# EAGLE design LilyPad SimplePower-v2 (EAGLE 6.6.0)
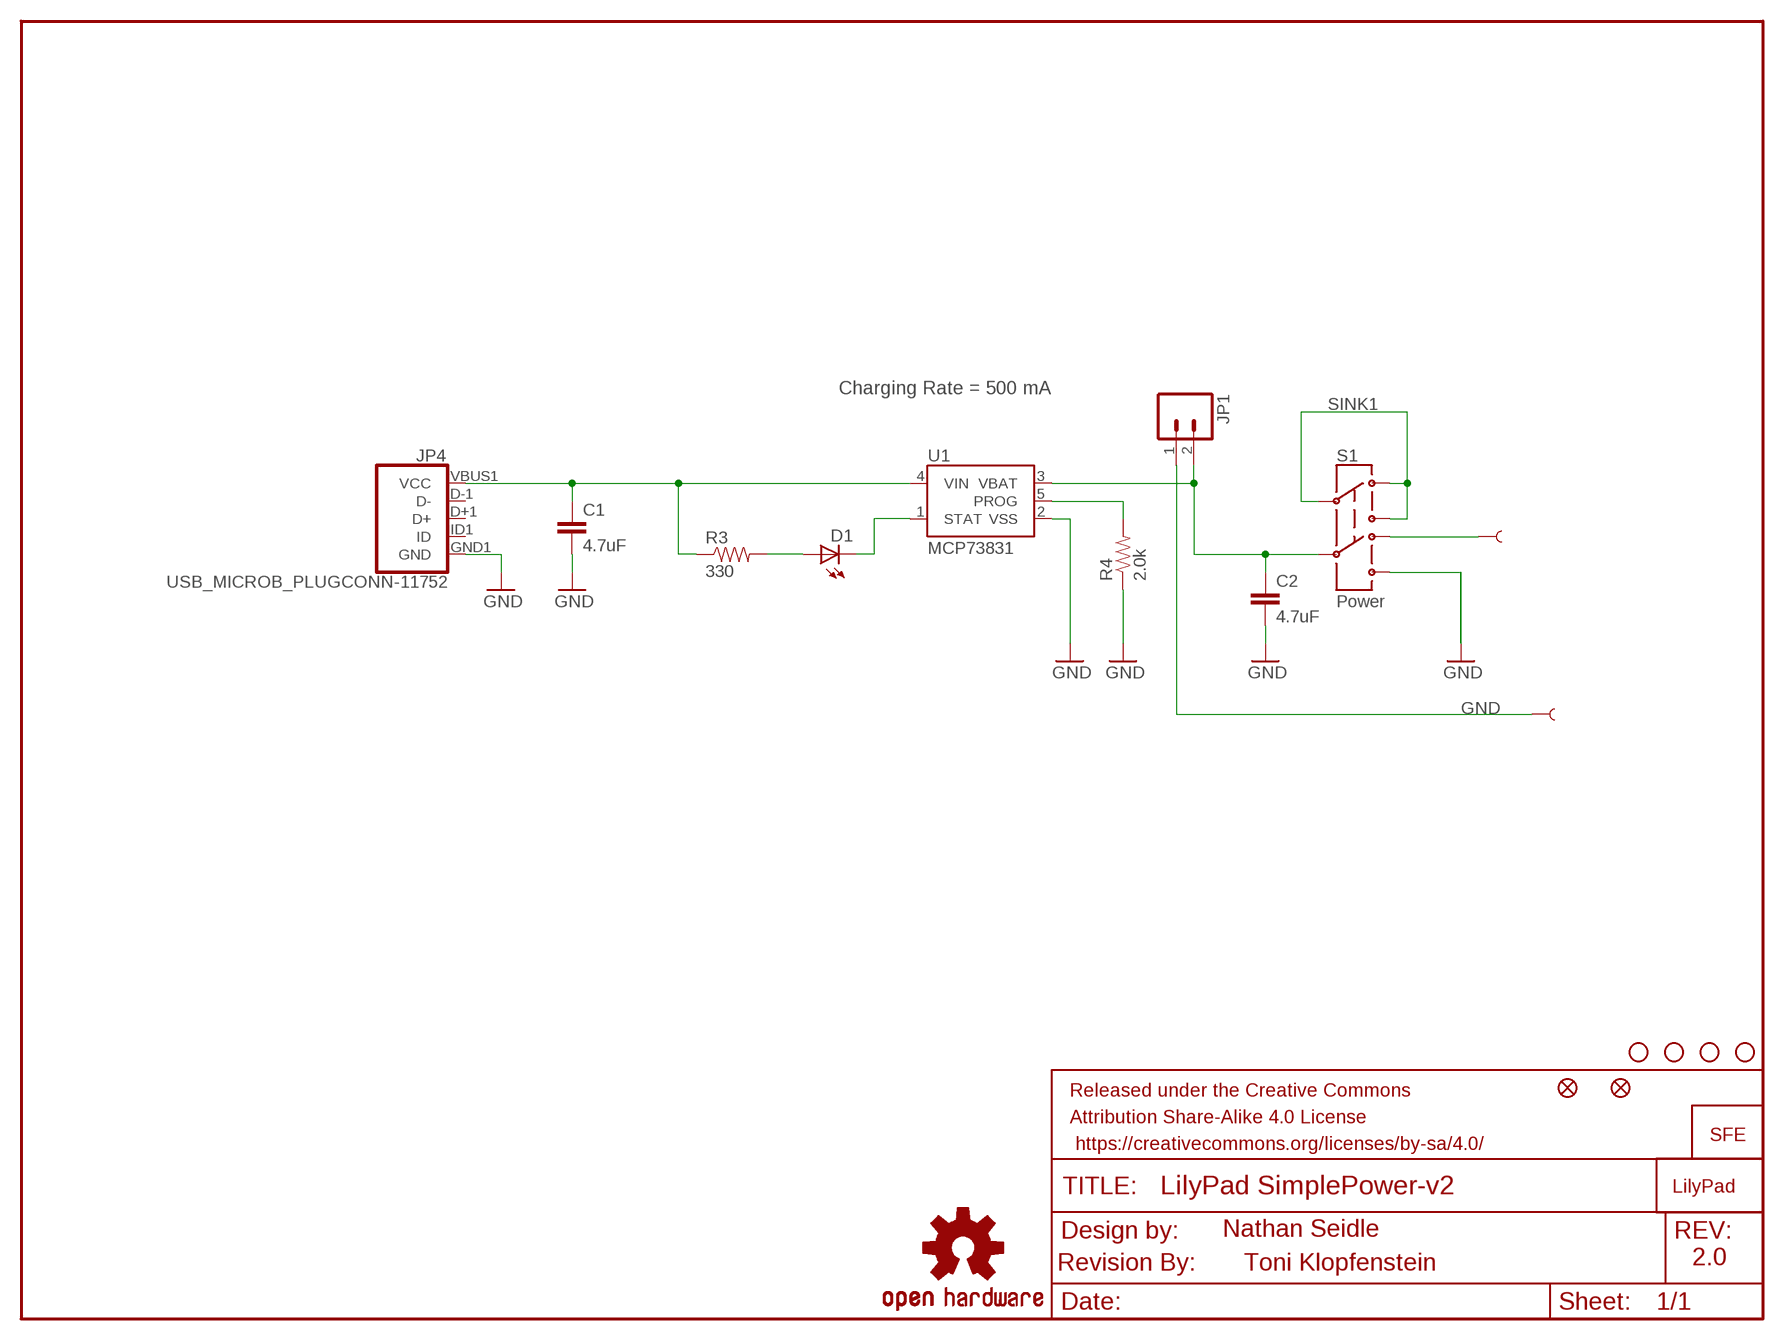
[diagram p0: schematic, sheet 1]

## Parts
C1  4.7uF  4.7UF-6.3V-10%(0603)0603  [0603-CAP]
C2  4.7uF  4.7UF-6.3V-10%(0603)0603  [0603-CAP]
D1  LED-YELLOW0603  [LED-0603]
FID1  FIDUCIAL1X2  [FIDUCIAL-1X2]
FID2  FIDUCIAL1X2  [FIDUCIAL-1X2]
FRAME1  FRAME-LETTER  [CREATIVE_COMMONS]
JP1  M02-JST-2MM-SMT  [JST-2-SMD]
JP3  LOGO-SFESK  [SFE-LOGO-FLAME]
JP4  USB_MICROB_PLUGCONN-11752  [USB-B-MICRO-SMD_V03]
R3  330  330OHM1/10W1%(0603)  [0603-RES]
R4  2.0k  2.0KOHM1/10W5%(0603)  [0603-RES]
S1  Power  SWITCH-DPDTSMD  [AYZ0202]
STANDOFF1  SEW-HOLE-NO-PAD  [SEW-HOLE-NO-PAD]
STANDOFF2  SEW-HOLE-NO-PAD  [SEW-HOLE-NO-PAD]
STANDOFF3  SEW-HOLE-NO-PAD  [SEW-HOLE-NO-PAD]
STANDOFF4  SEW-HOLE-NO-PAD  [SEW-HOLE-NO-PAD]
U1  MCP73831  [SOT23-5]
U$1  LOGO-LPLP  [LOGO-LILYPAD]
U$3  SEWTAP9  [PETAL-LONG-1-2SIDE]
U$4  SEWTAP9  [PETAL-LONG-1-2SIDE]
U$5  OSHW-LOGOS  [OSHW-LOGO-S]
U$6  REVISION  [REVISION]

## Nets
GND: C1.2 C2.2 JP1.1 JP4.GND1(GND) R4.1 S1.6 U1.2(VSS) U$3.1
N$1: C2.1 JP1.2 S1.5 U1.3(VBAT)
N$3: C1.1 JP4.VBUS1(VCC) R3.1 U1.4(VIN)
N$4: D1.C U1.1(STAT)
N$5: D1.A R3.2
N$6: S1.4 U$4.1
N$7: R4.2 U1.5(PROG)
SINK1: S1.1 S1.2 S1.3
Unconnected: JP4.D+1(D+) JP4.D-1(D-) JP4.ID1(ID)

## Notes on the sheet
- Charging Rate = 500 mA
- Nathan Seidle
- Toni Klopfenstein | 2.0

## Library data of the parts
C1 C2 = SparkFun-Capacitors:4.7UF-6.3V-10%(0603): CAP-08280; PROD_ID: CAP-08280
D1 = SparkFun-LED:LED-YELLOW: Yellow SMD LEDs; PROD_ID: DIO-09003
FID1 FID2 = SparkFun-Aesthetics:FIDUCIAL: Fiducial Alignment Points
FRAME1 = SparkFun-Aesthetics:FRAME-LETTER: Schematic Frame
JP1 = SparkFun:M02: Header 2
JP3 = SparkFun-Aesthetics:LOGO-SFE: Spark Fun Electronics PCB Logo
JP4 = SparkFun-Connectors:USB_MICROB_PLUG: USB Micro-B Plug Comes in a variety of packages. Check out Hirose's ZX-x0 line: http://www.hirose.co.jp/cataloge_hp/e24200011.pdf; PROD_ID: CONN-11752
R3 = SparkFun-Resistors:330OHM1/10W1%(0603): RES-00818; PROD_ID: RES-00818
R4 = SparkFun-Resistors:2.0KOHM1/10W5%(0603): RES-08296; PROD_ID: RES-08296
S1 = SparkFun:SWITCH-DPDT: DPDT Version of the COM-00597
STANDOFF1-STANDOFF4 = Local Library:SEW-HOLE-NO-PAD: #4 Stand Off
U1 = SparkFun-PowerIC:MCP73831: Miniature single cell, fully integrated Li-Ion, Li-polymer charge management controller http://ww1.microchip.com/downloads/en/DeviceDoc/21984a.pdf IC-09995; PROD_ID: IC-09995
U$1 = LilyPad-Wearables:LOGO-LP
U$3 U$4 = LilyPad-Wearables:SEWTAP
U$5 = SparkFun-Aesthetics:OSHW-LOGO: Open Source Hardware Logo This logo indicates the piece of hardware it is found on incorporates a OSHW license and/or adheres to the definition of open source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
U$6 = SparkFun-Aesthetics:REVISION

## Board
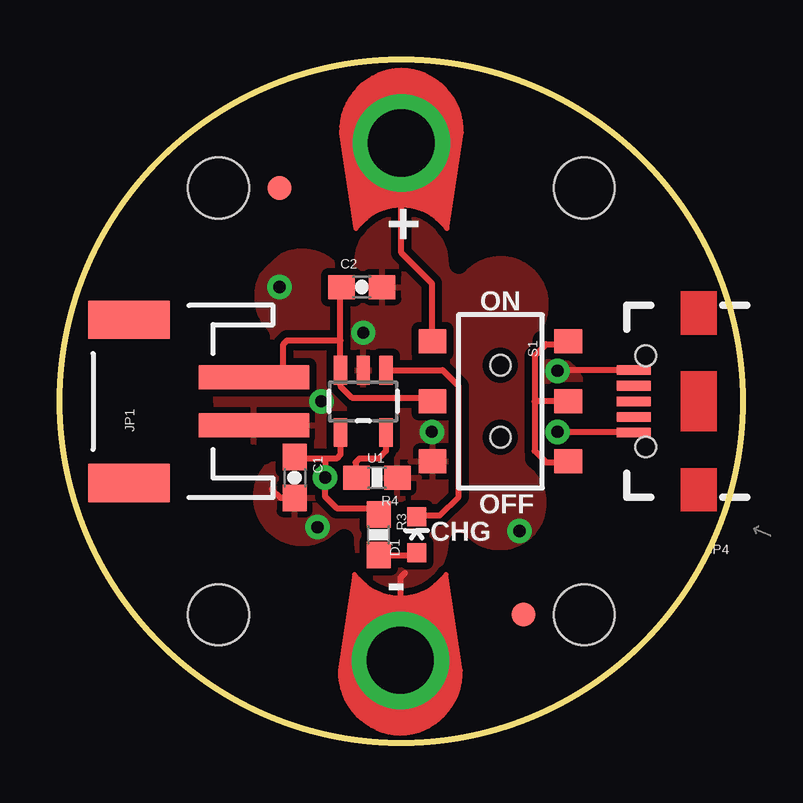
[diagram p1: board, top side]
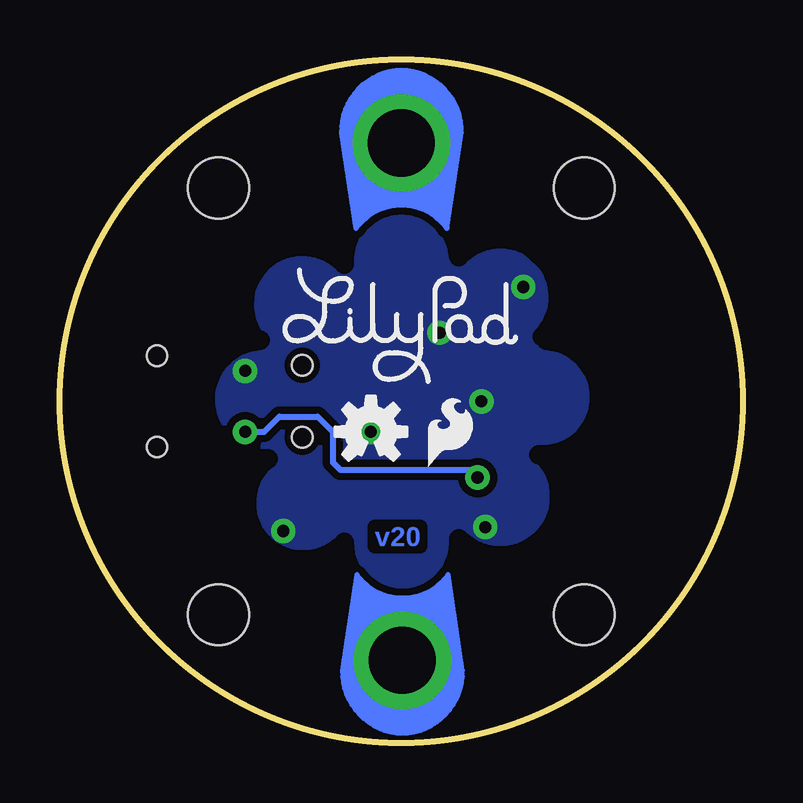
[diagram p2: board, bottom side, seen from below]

Size 28.45 x 28.45 mm. Coordinates in mm from the lower left corner, seen from the top.
Outline: circle at 14.22,14.22 radius 14.22
Copper layers (1*16): Top 0.035mm / dielectric 1.5mm / Bottom 0.035mm
Design rules "SparkFun-2-layer": minimum track width 7mil, minimum drill 15mil, track to track 8mil, track to pad 8mil, pad to pad 8mil, via to via 8mil, smd to smd 8mil, copper to edge 8mil, drill to drill 8mil, minimum pad ring 12mil, minimum via ring 10mil, stop-mask expansion 4mil, vias tented up to drill 20mil, thermal gap 10mil
tRestrict: area 2.9,2.9 to 25.6,25.6; 8 lines
bRestrict: area 2.9,2.9 to 25.6,25.6; 8 lines

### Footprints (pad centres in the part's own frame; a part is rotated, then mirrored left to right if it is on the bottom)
0603-CAP = smd 1.1 x 1: 1 -0.85,0; 2 0.85,0
LED-0603 = smd 0.8 x 0.8: A 0,-0.75; C 0,0.75
FIDUCIAL-1X2 = smd 1 x 1: 1 0,0
JST-2-SMD = smd 1 x 4.6: 1 -1,-3.7; 2 1,-3.7 | smd 1.6 x 3.4: NC1 -3.4,1.5; NC2 3.4,1.5
USB-B-MICRO-SMD_V03 = smd 1.4 x 0.4: D+1 2.7,0; D-1 2.7,0.65; GND1 2.7,-1.3; ID1 2.7,-0.65; VBUS1 2.7,1.3 | hole 0.85: 2.2,1.9; 2.2,-1.9
0603-RES = smd 1.1 x 1: 1 -0.85,0; 2 0.85,0
AYZ0202 = smd 1 x 1.15: 1 -2.5,2.825; 2 0,2.825; 3 2.5,2.825; 4 -2.5,-2.825; 5 0,-2.825; 6 2.5,-2.825 | hole 0.85: 1.5,0; -1.5,0
SEW-HOLE-NO-PAD = hole 2.54: 0,0
SOT23-5 = smd 0.55 x 1.2: 1 -0.95,-1.3; 2 0,-1.3; 3 0.95,-1.3; 4 0.95,1.3; 5 -0.95,1.3
PETAL-LONG-1-2SIDE = drill 2.794 pad 4.064: 1 0.03,0

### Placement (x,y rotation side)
C1  9.78,11.05 270 top
C2  12.57,18.99 0 top
D1  14.86,8.67 0 top
FID1  9.14,23.11 0 top
FID2  19.3,5.33 0 top
FRAME1  not placed on the board
JP1  4.38,14.22 90 top
JP3  13.11,11.53 0 bottom
JP4  26.61,14.22 180 top
R3  13.27,8.67 270 top
R4  13.21,11.05 180 top
S1  18.35,14.22 270 top
STANDOFF1  6.6,23.11 0 top
STANDOFF2  21.84,23.11 0 top
STANDOFF3  21.84,5.33 0 top
STANDOFF4  6.6,5.33 0 top
U1  12.64,14.22 180 top
U$1  14.22,17.72 0 bottom
U$3  14.18,3.4 90 top
U$4  14.22,25.02 270 top
U$5  15.49,12.95 0 bottom
U$6  not placed on the board

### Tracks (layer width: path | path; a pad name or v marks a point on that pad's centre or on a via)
GND  (via drill 0.51)
  Top 0.203: U$3.1 14.18,5.7
  Top 0.254: 14.22,5.49 14.22,5.65 | 14.22,5.81 14.22,5.97 | JP4.GND1 20.76,15.52 v20.73,15.49 | 14.38,7.08 14.18,6.88 14.18,5.92 14.06,5.81 | C1.2 9.2,10.2 8.83,10.57 | JP1.1 8.19,13.11 8.83,13.11 8.98,12.95 8.83,12.95 | 14.22,5.65 14.06,5.65 14.06,5.81 | 14.06,5.81 14.22,5.81 | 14.22,5.81 14.22,5.65 | 14.22,5.49 14.22,5.02 | 14.18,5.7 14.18,5.54 14.22,5.49
  Bottom 0.254: 15.81,13.91 15.49,13.59 v15.49,12.95
  other vias: 10.89,14.22 9.14,18.99 12.64,17.08 19.15,8.83 10.73,8.99
  pour Bottom (isolate 0.305): 0.25,28.19 0.25,0.25 28.19,0.25 28.19,28.19
  pour Top (isolate 0.305): 0.25,28.19 0.25,0.25 28.19,0.25 28.19,28.19
N$1
  Top 0.254: 15.21,13.91 S1.5 15.37,14.38 12.16,14.38 11.69,14.86 U1.3 11.69,16.76 | 11.69,16.76 11.69,18.95 C2.1 | JP1.2 9.25,15.22 9.3,15.18 9.3,16.61 9.46,16.76 11.69,16.76
N$3  (via drill 0.51)
  Top 0.254: v20.73,12.95 23.88,12.95 JP4.VBUS1 | U1.4 11.69,12 11.53,11.84 11.05,11.84 | 11.05,11.84 9.84,11.84 C1.1 | 11.05,11.84 v11.05,11.05 11.05,10.25 11.53,9.78 13.01,9.78 R3.1
  Bottom 0.254: v11.05,11.05 11.37,11.37 16.76,11.37 17.08,11.68 17.08,12.95 17.72,13.59 19.3,13.59 19.94,12.95 v20.73,12.95
N$4
  Top 0.254: U1.1 15.94,15.52 16.61,14.86 16.61,10.25 15.81,9.46 14.9,9.46 D1.C
N$5
  Top 0.254: R3.2 14.76,7.82 D1.A
N$6
  Top 0.254: U$4.1 14.22,20.41 15.49,19.14 15.49,16.76 S1.4
N$7
  Top 0.254: U1.5 13.59,12.16 13.27,11.84 12.48,11.84 12.32,11.68 12.32,11.09 R4.2
SINK1
  Top 0.254: S1.3 21.14,11.68 20.26,11.68 19.78,12.16 19.78,14.22 | S1.1 21.06,16.61 20.26,16.61 19.78,16.13 19.78,14.22 | S1.2 19.78,14.22

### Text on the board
Bottom: v20
tPlace: + | ON | OFF | CHG | -
tDocu: N. Seidle | Toni Klopfenstein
